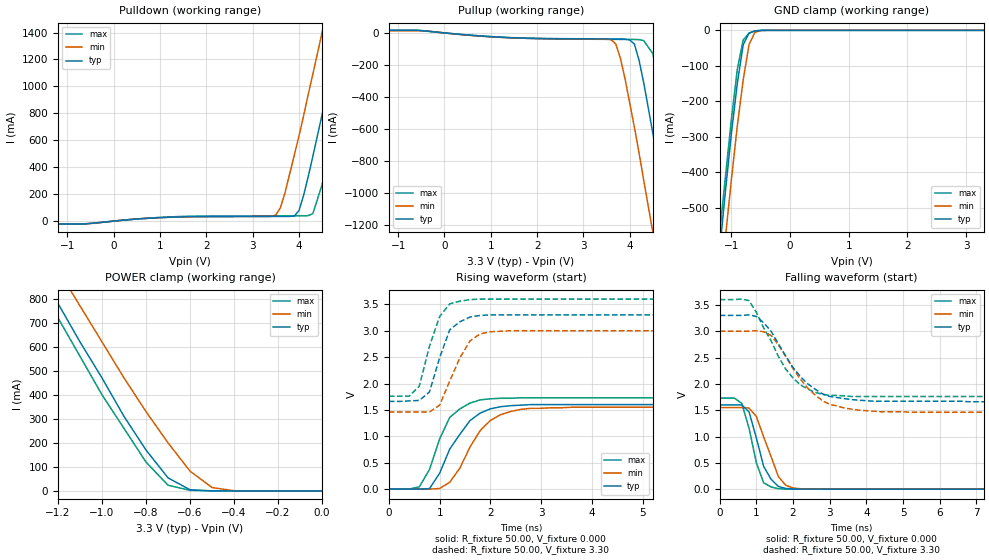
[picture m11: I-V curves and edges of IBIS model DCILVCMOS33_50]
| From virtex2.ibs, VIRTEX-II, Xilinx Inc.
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|   Model DCILVCMOS33_50
[Model]   DCILVCMOS33_50
Model_type   I/O
Polarity   Non-Inverting
Enable   Active-Low
Vinh = 2.0V
Vinl = 0.8V
Vmeas =   1.65V
Cref =  35.00pF
Rref =   1.00M
Vref =  0.000V
C_comp   7.00pF   6.00pF   8.00pF
[Temperature Range]   25.00   100.00   0.000
[Voltage Range]   3.30V   3.00V   3.60V
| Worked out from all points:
|   slope of the pulldown table from 0 to 0.495 V, typ, clamps not added: 32.3 ohm
|   slope of the pullup table from 0 to 0.495 V, typ, clamps not added: 38.4 ohm
|   GND clamp passes 1 mA (typ) near -0.57 V on its own axis
|   POWER clamp passes 1 mA (typ) near -0.52 V on its own axis
|   rising waveform, R_fixture 50.00, V_fixture 0.000: 20-80 % time 576ps typ, 604ps min, 445ps max; typ from 0 V to 1.6 V
|   rising waveform, R_fixture 50.00, V_fixture 3.30: 20-80 % time 336ps typ, 449ps min, 340ps max; typ from 1.66 V to 3.3 V
|   falling waveform, R_fixture 50.00, V_fixture 0.000: 20-80 % time 416ps typ, 491ps min, 376ps max; typ from 1.6 V to 0 V
|   falling waveform, R_fixture 50.00, V_fixture 3.30: 20-80 % time 1ns typ, 996ps min, 893ps max; typ from 3.3 V to 1.66 V
[Pulldown]
| voltage   I(typ)   I(min)   I(max)
-3.3V     -21.65mA   -19.86mA   -21.8mA
3.5V      34.6mA     44.62mA    38.71mA
3.6V      34.64mA    100mA      38.74mA
3.7V      34.69mA    210mA      38.78mA
4V        77.2mA     630mA      38.89mA
4.2V      330mA      940mA      40.79mA
4.3V      480mA      1.09A      55.46mA
4.5V      790mA      1.4A       270mA
4.9V      1.44A      2.02A      890mA
5.1V      1.77A      2.33A      1.22A
5.3V      2.1A       2.65A      1.55A
6.6V      4.27A      4.71A      3.71A
[Pullup]
| voltage   I(typ)   I(min)   I(max)
-3.3V     16.86mA    13.72mA    16.49mA
3.6V      -37.66mA   -42.86mA   -40.19mA
3.7V      -37.77mA   -69.63mA   -40.32mA
3.8V      -37.96mA   -160mA     -40.45mA
4.1V      -69.61mA   -590mA     -40.87mA
4.3V      -310mA     -920mA     -47.66mA
4.5V      -630mA     -1.25A     -130mA
4.7V      -970mA     -1.58A     -420mA
4.9V      -1.31A     -1.92A     -750mA
5.1V      -1.66A     -2.26A     -1.09A
5.3V      -2.01A     -2.61A     -1.44A
6.6V      -4.31A     -4.84A     -3.74A
[GND_clamp]
| voltage   I(typ)   I(min)   I(max)
-3.3V     -4.3A      -4.31A     -4.26A
-1.2V     -620mA     -740mA     -570mA
-1.1V     -450mA     -580mA     -410mA
-1V       -290mA     -420mA     -250mA
-900mV    -150mA     -270mA     -110mA
-800mV    -41.03mA   -140mA     -27.28mA
-700mV    -7.6mA     -40.21mA   -8.18mA
-600mV    -1.42mA    -5.61mA    -1.62mA
-500mV    -130uA     -670uA     -130uA
3.3V      67.85pA    43.48uA    45.6pA
[POWER_clamp]
| voltage   I(typ)   I(min)   I(max)
-3.3V     4.25A      4.22A      4.2A
-1.3V     940mA      1.07A      880mA
-1.2V     780mA      920mA      720mA
-1.1V     620mA      770mA      560mA
-1V       470mA      620mA      400mA
-900mV    310mA      470mA      260mA
-800mV    170mA      330mA      120mA
-700mV    54.34mA    200mA      23.62mA
-600mV    4.76mA     82.21mA    2.52mA
-500mV    280uA      14.02mA    260uA
-400mV    16.9uA     860uA      14.85uA
0V        67.85pA    2.04nA     61.89pA
[Ramp]
| variable   typ   min   max
dV/dt_r   0.96/0.52n   0.93/0.57n   1.04/0.43n
dV/dt_f   0.98/0.99n   0.92/0.98n   1.11/0.83n
R_load = 50.00
[Rising Waveform]
R_fixture = 50.00
V_fixture = 0.000
| time   V(typ)   V(min)   V(max)
0s        0V         0V         0V
600ps     -2.17mV    46.96uV    42.03mV
800ps     8.09mV     -900uV     370mV
1ns       300mV      10.79mV    950mV
1.2ns     760mV      130mV      1.36V
1.6ns     1.3V       800mV      1.63V
1.8ns     1.44V      1.11V      1.69V
2.2ns     1.56V      1.41V      1.72V
2.8ns     1.6V       1.53V      1.73V
10ns      1.6V       1.55V      1.73V
[Rising Waveform]
R_fixture = 50.00
V_fixture = 3.30
V_fixture_min = 3.00
V_fixture_max = 3.60
| time   V(typ)   V(min)   V(max)
0s        1.66V      1.46V      1.76V
400ps     1.67V      1.46V      1.76V
600ps     1.68V      1.46V      1.95V
800ps     1.84V      1.46V      2.71V
1ns       2.49V      1.59V      3.27V
1.2ns     3.02V      2.05V      3.51V
1.4ns     3.17V      2.49V      3.56V
1.6ns     3.26V      2.81V      3.59V
2ns       3.3V       2.98V      3.6V
10ns      3.3V       3V         3.6V
[Falling Waveform]
R_fixture = 50.00
V_fixture = 0.000
| time   V(typ)   V(min)   V(max)
0s        1.6V       1.55V      1.73V
600ps     1.6V       1.55V      1.63V
800ps     1.47V      1.54V      1.16V
1ns       970mV      1.38V      500mV
1.2ns     430mV      990mV      120mV
1.4ns     190mV      620mV      42.64mV
1.6ns     52.11mV    240mV      8.09mV
1.8ns     12.91mV    74.61mV    2.16mV
2.2ns     1.53mV     6.55mV     590uV
10ns      2.72uV     3.42uV     1.92uV
[Falling Waveform]
R_fixture = 50.00
V_fixture = 3.30
V_fixture_min = 3.00
V_fixture_max = 3.60
| time   V(typ)   V(min)   V(max)
0s        3.3V       3V         3.6V
800ps     3.31V      3V         3.58V
1ns       3.28V      3.01V      3.36V
1.4ns     3V         2.92V      2.82V
1.8ns     2.53V      2.52V      2.28V
2ns       2.31V      2.29V      2.11V
2.4ns     2V         1.92V      1.9V
2.8ns     1.81V      1.68V      1.8V
4.4ns     1.67V      1.47V      1.76V
10ns      1.66V      1.46V      1.76V
